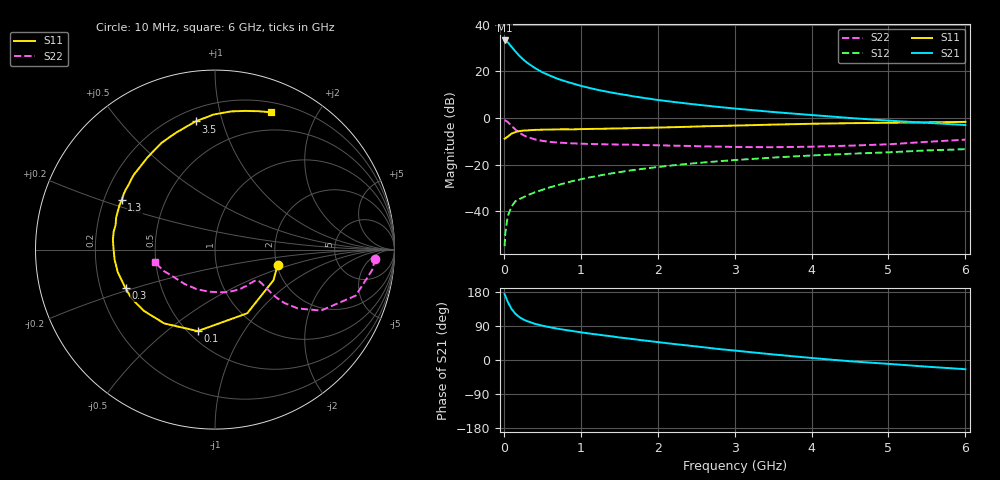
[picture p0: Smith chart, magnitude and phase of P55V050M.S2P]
! SIEMENS Small Signal Semiconductors
! BFP183
! Si NPN RF Bipolar Junction Transistor in SOT143
! VCE = 5 V  IC = 50 mA
! Common Emitter S-Parameters:  March  1996
# GHz  S  MA  R  50
!  f  S11  S21  S12  S22
! GHz  MAG  ANG  MAG  ANG  MAG  ANG  MAG  ANG
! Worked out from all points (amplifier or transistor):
!   36 points, 10 MHz to 6 GHz, reference 50 ohm
!   highest |S21| = 33.2 dB at 10 MHz (marker M1)
!   |S21| within 3 dB of that: start of sweep to 107.3 MHz
!   unconditionally stable (mu >= 1): start of sweep to 11.18 MHz; 439.3 MHz to end of sweep
!   at 250 MHz: K = 0.76, MSG = 29.6 dB, |S12| = -34.0 dB
!   at 1.4 GHz: K = 1.27, MAG = 14.2 dB, |S12| = -23.7 dB
!   at 6 GHz: K = 1.01, MAG = 4.4 dB, |S12| = -13.4 dB
!   S11 on the Smith chart (normalised r, x): 10 MHz: 2.02, -0.40; 100 MHz: 0.56, -0.64; 300 MHz: 0.31, -0.19; 1.3 GHz: 0.27, +0.23; 3.5 GHz: 0.28, +0.82; 6 GHz: 0.30, +1.44
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0.01  0.3598 -13.9  45.8 174.2  0.0018 80.3  0.8933 -3.3
0.02  0.3677 -27.7  45.56 169.2  0.0035 77.6  0.8837 -7.3
0.05  0.3977 -63.2  42.05 153.7  0.0078 72.9  0.825 -18.1
0.1  0.4642 -102.0  33.52 134.7  0.0127 57.0  0.6815 -29.9
0.15  0.4992 -124.5  26.69 122.0  0.0165 53.0  0.566 -35.4
0.2  0.5228 -139.2  21.69 113.5  0.0183 51.7  0.4866 -37.6
0.25  0.5381 -149.2  18.01 107.3  0.0199 52.1  0.4329 -38.0
0.3  0.543 -156.6  15.43 102.8  0.0219 52.4  0.3946 -37.6
0.4  0.556 -166.9  11.88 95.7  0.0255 54.4  0.35 -36.7
0.5  0.5624 -174.5  9.554 90.6  0.0289 55.9  0.3239 -36.0
0.6  0.5654 179.5  8.079 86.3  0.0328 57.1  0.3083 -35.7
0.7  0.5714 174.6  6.912 82.6  0.0366 59.0  0.2984 -35.8
0.8  0.5733 170.0  6.109 79.2  0.0405 59.5  0.2919 -36.3
1.1  0.5823 158.3  4.458 70.2  0.0529 60.1  0.2784 -39.5
1.3  0.5887 151.9  3.767 64.9  0.061 59.5  0.274 -42.6
1.7  0.6099 139.6  2.888 54.7  0.0776 57.1  0.2672 -50.0
2.2  0.6362 126.4  2.218 42.5  0.097 53.0  0.2556 -61.0
2.8  0.6755 112.1  1.72 28.8  0.1188 47.1  0.2441 -77.1
3.5  0.7224 98.6  1.345 14.7  0.1421 40.6  0.2372 -98.4
4.5  0.7752 83.4  1.001 -3.3  0.1715 30.9  0.2559 -131.5
5.5  0.8076 72.7  0.789 -17.6  0.2022 22.5  0.3088 -157.2
6  0.826 67.9  0.708 -24.3  0.215 17.6  0.3439 -168.3
